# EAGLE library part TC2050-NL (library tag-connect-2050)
TAG-CONNECT ISP Connector Manufacturer: Tag-Connect Cable for easy In-Circuit PCB Programming. Designed for JTAG 10 pin, suitable for many others. Pin Connection for TC2050 NL. PADDescription 1VTREF 2TMS 3GND 4TCK 5NC 6TDO 7RTCK 8TDI 9!TRST 10RESET ©2009 ROFA.cz Modified 7/2011 by Tim McCarthy-Smith VIDA Products INC
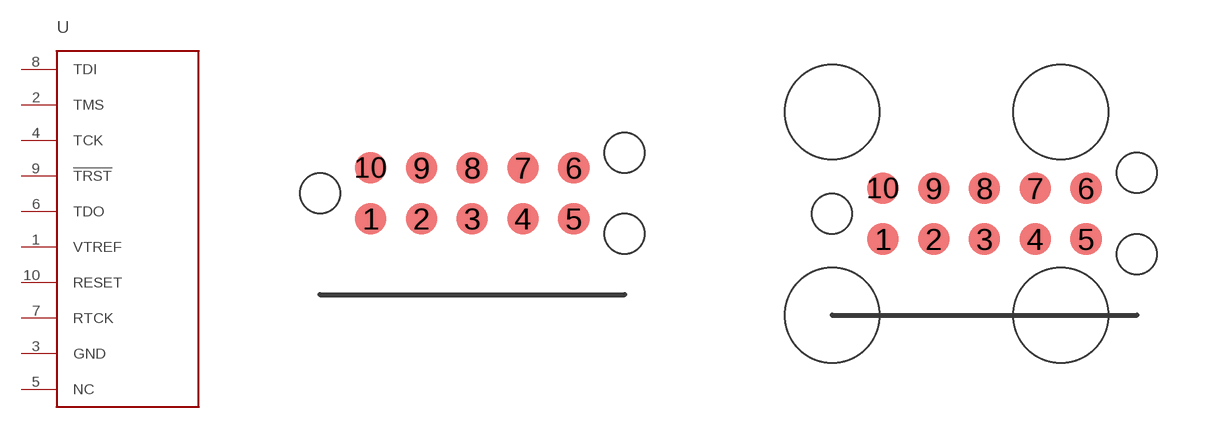
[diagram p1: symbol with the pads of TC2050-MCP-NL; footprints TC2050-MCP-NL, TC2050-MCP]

Designator prefix -

## TC2050-NL-MCP-NL  [TC2050-MCP-NL]
1  VTREF
2  TMS
3  GND
4  TCK
5  NC
6  TDO
7  RTCK
8  TDI
9  !TRST
10  RESET

## TC2050-NL  [TC2050-MCP]
Pads as for TC2050-MCP-NL

## Footprint TC2050-MCP-NL (pad centres in mm)
TAG-CONNECT ISP Connector Manufacturer: Tag-Connect Cable for easy In-Circuit PCB Programming. Designed for Standard JTAG 10 Pin, suitable for many others. Footprint for TC2050 NL PADDescription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
smd 0.787 x 0.787: 1 1.27,-0.635; 2 2.54,-0.635; 3 3.81,-0.635; 4 5.08,-0.635; 5 6.35,-0.635; 6 6.35,0.635; 7 5.08,0.635; 8 3.81,0.635; 9 2.54,0.635; 10 1.27,0.635
hole 1 at 0,0
hole 1 at 7.62,-1.016
hole 1 at 7.62,1.016

## Footprint TC2050-MCP (pad centres in mm)
TAG-CONNECT ISP Connector Manufacturer: Tag-Connect Cable for easy In-Circuit PCB Programming. Designed for Standard JTAG 10 Pin, suitable for many others. Footprint for TC2050 NL PADDescription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
smd 0.787 x 0.787: 1 1.27,-0.635; 2 2.54,-0.635; 3 3.81,-0.635; 4 5.08,-0.635; 5 6.35,-0.635; 6 6.35,0.635; 7 5.08,0.635; 8 3.81,0.635; 9 2.54,0.635; 10 1.27,0.635
hole 1 at 0,0
hole 1 at 7.62,-1.016
hole 1 at 7.62,1.016
hole 2.375 at 0,2.54
hole 2.375 at 0,-2.54
hole 2.375 at 5.715,2.54
hole 2.375 at 5.715,-2.54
